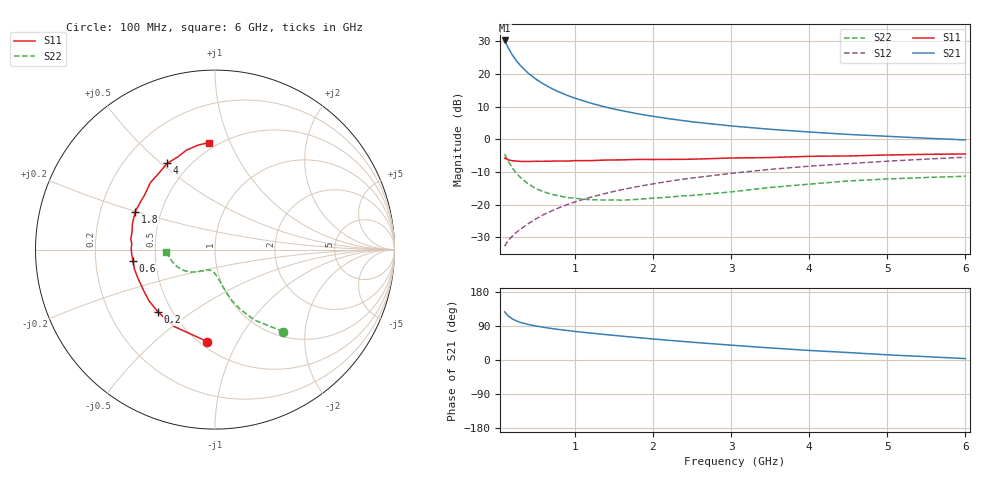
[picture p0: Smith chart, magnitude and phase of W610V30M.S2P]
! SIEMENS Small Signal Semiconductors
! BFR193W
! Si NPN RF Bipolar Junction Transistor in SOT323
! VCE = 10 V  IC = 30 mA
! Common Emitter S-Parameters:  September  1992
# GHz  S  MA  R  50
!  f  S11  S21  S12  S22
! GHz  MAG  ANG  MAG  ANG  MAG  ANG  MAG  ANG
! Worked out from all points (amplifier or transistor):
!   28 points, 100 MHz to 6 GHz, reference 50 ohm
!   highest |S21| = 30.2 dB at 100 MHz (marker M1)
!   |S21| within 3 dB of that: start of sweep to 163.8 MHz
!   unconditionally stable (mu >= 1): 707.5 MHz to 2.679 GHz
!   at 300 MHz: K = 0.82, MSG = 25.1 dB, |S12| = -27.5 dB
!   at 1.5 GHz: K = 1.03, MAG = 11.5 dB, |S12| = -15.9 dB
!   at 6 GHz: K = 0.91, MSG = 2.6 dB, |S12| = -5.5 dB
!   S11 on the Smith chart (normalised r, x): 100 MHz: 0.55, -0.76; 200 MHz: 0.42, -0.38; 600 MHz: 0.37, -0.06; 1.8 GHz: 0.35, +0.20; 4 GHz: 0.38, +0.52; 6 GHz: 0.45, +0.84
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0.1  0.5145 -94.7  32.42 127.1  0.0233 58.8  0.5933 -50.3
0.15  0.4851 -117.9  24.47 115.6  0.0289 57.0  0.4528 -60.5
0.2  0.4708 -132.2  19.39 108.2  0.0332 57.8  0.365 -66.8
0.25  0.4656 -142.1  15.94 103.3  0.0378 58.9  0.3029 -71.3
0.3  0.4588 -149.6  13.52 99.4  0.0421 60.8  0.2637 -73.9
0.4  0.4584 -160.2  10.3 93.8  0.0512 63.7  0.2091 -78.2
0.5  0.4619 -166.9  8.326 89.7  0.0607 66.0  0.1773 -81.2
0.6  0.4616 -172.4  6.984 86.3  0.0708 67.2  0.1578 -84.6
0.7  0.4643 -176.6  5.991 83.1  0.0804 68.2  0.1448 -86.8
0.8  0.4671 179.3  5.278 80.4  0.0904 68.6  0.1367 -89.5
0.9  0.465 175.8  4.7 77.9  0.1005 68.9  0.129 -91.3
1  0.4726 173.1  4.264 75.4  0.1104 68.9  0.1257 -93.5
1.2  0.4729 167.5  3.579 71.1  0.1304 68.5  0.1193 -98.9
1.5  0.4838 161.0  2.905 65.0  0.1599 67.3  0.1187 -105.6
1.8  0.4928 154.7  2.464 59.2  0.1895 65.5  0.121 -111.2
2.2  0.4931 146.8  2.068 52.0  0.228 63.0  0.1307 -116.9
3  0.5185 134.0  1.603 39.2  0.302 56.9  0.1574 -128.1
3.5  0.5271 126.9  1.424 31.8  0.3474 52.8  0.1837 -137.0
4  0.5495 119.0  1.295 25.2  0.3884 48.5  0.2066 -145.4
4.5  0.5569 111.6  1.188 19.7  0.4249 44.5  0.2309 -155.4
5.5  0.5893 99.4  1.039 8.8  0.4986 36.6  0.2611 -172.1
6  0.5974 93.4  0.979 3.7  0.5333 32.4  0.273 -176.7
